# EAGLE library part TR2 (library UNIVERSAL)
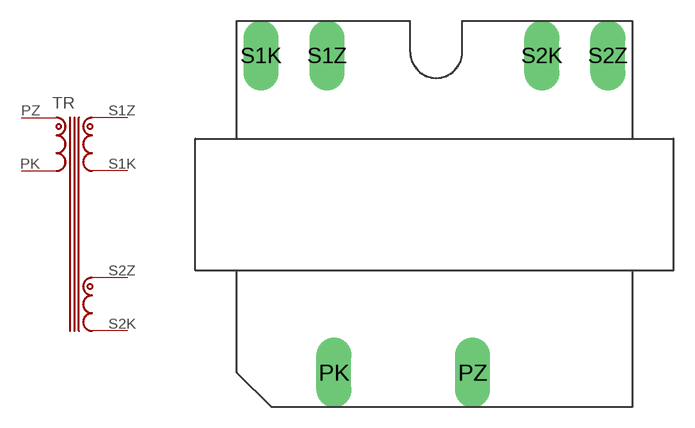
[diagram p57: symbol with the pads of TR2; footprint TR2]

Designator prefix TR

## TR2  [TR2]
PK  PK
PZ  PZ
S1K  S1K
S1Z  S1Z
S2K  S2K
S2Z  S2Z

## Footprint TR2 (pad centres in mm)
drill 0.8 pad 2.54 long: PK 7,3.135; PZ 17,3.135; S1K 1.75,26; S1Z 6.5,26; S2K 22,26; S2Z 26.75,26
